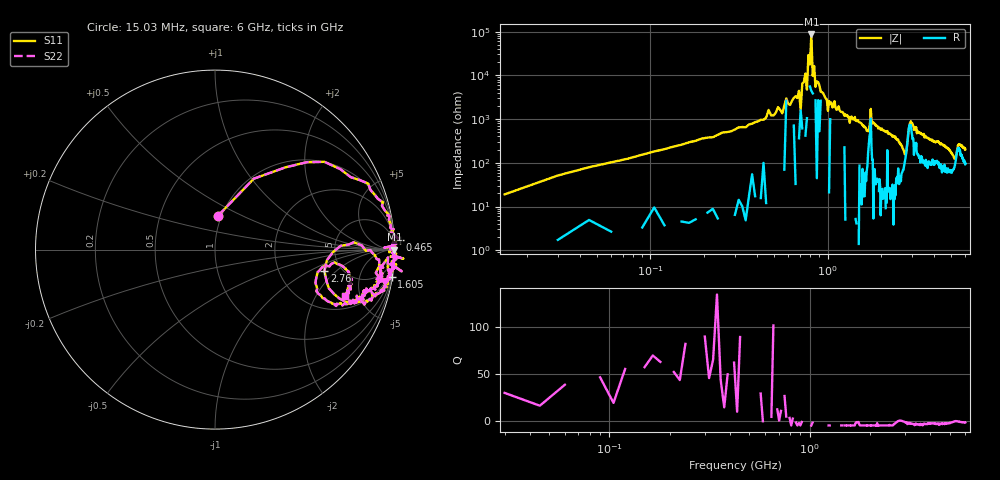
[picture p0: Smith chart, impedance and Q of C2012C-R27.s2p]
!	Network	Analyzer	HP8753E.07.74:	Oct	30	2002	Serial	No.	JP38451487
!	Hewlett-Packard
!	7	Sep	2009	12:22:38
!	Frequency	S11	S21	S12	S22
#	HZ	S	RI	R	50
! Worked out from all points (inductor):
!   400 points, 15.03 MHz to 6 GHz, reference 50 ohm
!   read as one part in series: L = 268 nH near 45.03 MHz
!   highest |Z| = 86.1 kohm at 810 MHz (marker M1)
!   self-resonance near 570 MHz
!   S11 on the Smith chart (normalised r, x): 15.03 MHz: 0.96, +0.38; 465 MHz: -17, +28; 1.605 GHz: 0, -13; 2.76 GHz: 3.70, -1.42; 6 GHz: 2.89, -3.60
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1.502992e7  0.0172 0.189  0.983 -0.189  0.983 -0.189  0.0172 0.189
1.350293e8  0.854 0.368  0.146 -0.368  0.146 -0.368  0.854 0.368
4.650277e8  1.03 0.0543  -0.0335 -0.0543  -0.0335 -0.0543  1.03 0.0543
6.900266e8  0.998 0.0224  0.00235 -0.0224  0.00235 -0.0224  0.998 0.0224
7.050265e8  0.943 0.0107  0.0574 -0.0107  0.0574 -0.0107  0.943 0.0107
7.500262e8  1 0.00909  0.000428 -0.00909  0.000428 -0.00909  1 0.00909
7.650262e8  0.995 0.0205  0.00513 -0.0205  0.00513 -0.0205  0.995 0.0205
7.800261e8  1 0.00336  -0.00067 -0.00336  -0.00067 -0.00336  1 0.00336
7.95026e8  0.998 0.00534  0.0018 -0.00534  0.0018 -0.00534  0.998 0.00534
8.10026e8  1 -0.00116  6.1e-05 0.00116  6.1e-05 0.00116  1 -0.00116
8.250259e8  0.996 0.00934  0.00415 -0.00934  0.00415 -0.00934  0.996 0.00934
8.400258e8  1 -0.0061  -6e-05 0.0061  -6e-05 0.0061  1 -0.0061
8.550257e8  0.991 -0.0157  0.00922 0.0157  0.00922 0.0157  0.991 -0.0157
1.020025e9  0.998 -0.0385  0.0018 0.0385  0.0018 0.0385  0.998 -0.0385
1.605022e9  0.984 -0.152  0.0165 0.152  0.0165 0.152  0.984 -0.152
1.755021e9  0.964 -0.0434  0.036 0.0434  0.036 0.0434  0.964 -0.0434
2.01002e9  0.967 -0.163  0.0334 0.163  0.0334 0.163  0.967 -0.163
2.760016e9  0.61 -0.118  0.39 0.118  0.39 0.118  0.61 -0.118
3.015015e9  0.937 -0.1  0.0629 0.1  0.0629 0.1  0.937 -0.1
4.00501e9  0.841 -0.242  0.159 0.242  0.159 0.242  0.841 -0.242
5.010005e9  0.678 -0.302  0.322 0.302  0.322 0.302  0.678 -0.302
6e9  0.723 -0.256  0.277 0.256  0.277 0.256  0.723 -0.256
